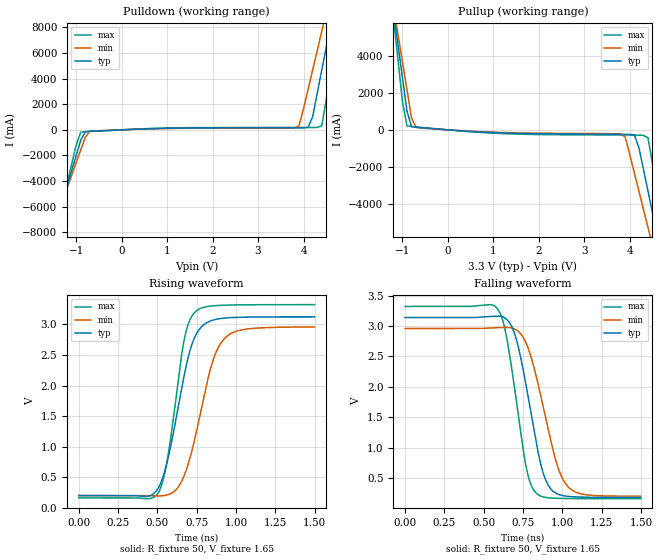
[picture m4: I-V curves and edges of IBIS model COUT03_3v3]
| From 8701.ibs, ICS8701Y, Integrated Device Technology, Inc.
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[Model] COUT03_3v3
Model_type   Output
Polarity   Non-Inverting
|   typ   min   max
C_comp   2pF   1.5pF   2.5pF
Vmeas = 1.65V
Rref = 50
Cref = 0
Vref = 1.65V
|   typ   min   max
[Voltage range]   3.3V   3.135V   3.465V
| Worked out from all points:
|   slope of the pulldown table from 0 to 0.495 V, typ, clamps not added: 6.88 ohm
|   slope of the pullup table from 0 to 0.495 V, typ, clamps not added: 5.83 ohm
|   rising waveform, R_fixture 50, V_fixture 1.65: 20-80 % time 138ps typ, 153ps min, 103ps max; typ from 0.197 V to 3.12 V
|   falling waveform, R_fixture 50, V_fixture 1.65: 20-80 % time 129ps typ, 153ps min, 108ps max; typ from 3.14 V to 0.181 V
[Pulldown]
|Voltage   I (typ)   I (min)   I (max)
-3.3V     -29.26A    -25.28A    -35.95A
-1.5V     -7.949A    -7.508A    -8.752A
-900mV    -829.9mA   -1.575A    -187.1mA
-700mV    -111.2mA   -118.1mA   -127.5mA
3.9V      159.4mA    311mA      182.9mA
4.1V      184.8mA    3.152A     184mA
4.2V      1.015A     4.66A      185mA
4.4V      4.637A     7.679A     308.5mA
4.6V      8.262A     10.7A      4.646A
4.7V      10.08A     12.21A     6.964A
4.8V      11.89A     13.72A     9.282A
6.6V      44.81A     41.14A     51.33A
[Pullup]
|Voltage   I (typ)   I (min)   I (max)
-3.3V     44.73A     38.61A     55.03A
-1.2V     6.49A      6.732A     6.202A
-1.1V     4.667A     5.214A     3.875A
-900mV    1.021A     2.176A     220.8mA
-700mV    135.9mA    139mA      157.7mA
3.8V      -238.9mA   -217.3mA   -279.5mA
4.1V      -276.1mA   -2.314A    -283.5mA
4.3V      -2.128A    -4.28A     -299.6mA
4.4V      -3.308A    -5.264A    -428.8mA
4.6V      -5.67A     -7.233A    -3.347A
4.8V      -8.032A    -9.203A    -6.363A
6.6V      -29.3A     -26.93A    -33.51A
[Ramp]
|   typ   min   max
dV/dt_r   2.352/0.212n   2.212/0.239n   2.54/0.159n
dV/dt_f   2.386/0.194n   2.222/0.231n   2.553/0.161n
R_load =   50.0000
[Rising Waveform]
R_fixture = 50
V_fixture = 1.65   |Vcc_typ
V_fixture_min = 1.5675 |Vcc_min
V_fixture_max = 1.7325 |Vcc_max
C_fixture = 0.0p
| Time   typ   min   max
0s        197mV      199.5mV    160.8mV
432.4ps   184.5mV    199.7mV    147.5mV
504.5ps   320.1mV    192.6mV    238.9mV
564.6ps   776.6mV    210.6mV    813.6mV
672.7ps   2.199V     544.3mV    2.782V
704.2ps   2.549V     791.9mV    3.061V
746.2ps   2.838V     1.226V     3.219V
849.9ps   3.068V     2.384V     3.303V
936.9ps   3.106V     2.795V     3.316V
1.498ns   3.124V     2.959V     3.323V
[Falling Waveform]
R_fixture = 50
V_fixture = 1.65   |Vcc_typ
V_fixture_min = 1.5675 |Vcc_min
V_fixture_max = 1.7325 |Vcc_max
C_fixture = 0.0p
| Time   typ   min   max
0s        3.141V     2.96V      3.323V
590.1ps   3.164V     2.975V     3.274V
638.1ps   3.128V     2.978V     2.911V
702.7ps   2.826V     2.944V     1.865V
774.8ps   1.952V     2.69V      623.4mV
839.3ps   1.017V     2.115V     239.2mV
912.9ps   372.3mV    1.274V     174.9mV
974.5ps   232.7mV    658.9mV    166.1mV
1.035ns   198.8mV    363.8mV    163.3mV
1.498ns   180.8mV    200.6mV    160.8mV
